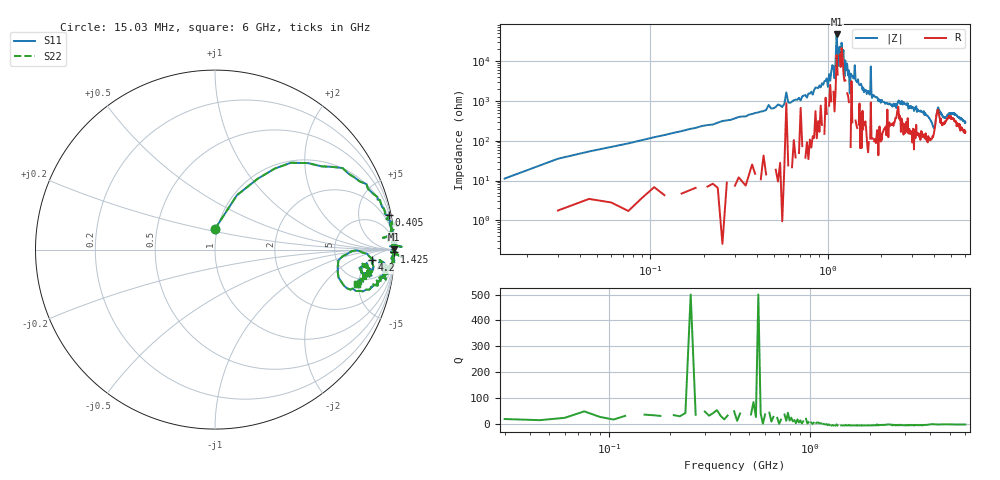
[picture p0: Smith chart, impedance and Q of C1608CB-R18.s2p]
!	Network	Analyzer	HP8753E.07.74:	Oct	30	2002	Serial	No.	JP38451487
!	Hewlett-Packard
!	7	Sep	2009	10:03:13
!	Frequency	S11	S21	S12	S22
#	HZ	S	RI	R	50
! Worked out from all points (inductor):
!   400 points, 15.03 MHz to 6 GHz, reference 50 ohm
!   read as one part in series: L = 184 nH near 45.03 MHz
!   highest |Z| = 45.7 kohm at 1.125 GHz (marker M1)
!   self-resonance near 1.185 GHz
!   S11 on the Smith chart (normalised r, x): 15.03 MHz: 0.97, +0.22; 405 MHz: 1, +10; 1.425 GHz: open; 4.2 GHz: 12, -6; 6 GHz: 4.26, -4.71
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1.502992e7  -0.00146 0.113  1 -0.113  1 -0.113  -0.00146 0.113
9.002955e7  0.518 0.482  0.482 -0.482  0.482 -0.482  0.518 0.482
4.05028e8  0.967 0.191  0.0333 -0.191  0.0333 -0.191  0.967 0.191
1.020025e9  0.996 0.0209  0.00382 -0.0209  0.00382 -0.0209  0.996 0.0209
1.095025e9  0.995 0.0268  0.00473 -0.0268  0.00473 -0.0268  0.995 0.0268
1.125024e9  0.999 0.00208  0.000672 -0.00208  0.000672 -0.00208  0.999 0.00208
1.155024e9  1 0.0134  3.1e-05 -0.0134  3.1e-05 -0.0134  1 0.0134
1.185024e9  0.986 0.000274  0.0139 -0.000274  0.0139 -0.000274  0.986 0.000274
1.200024e9  0.997 -0.00235  0.00262 0.00235  0.00262 0.00235  0.997 -0.00235
1.245024e9  0.98 -0.0148  0.0198 0.0148  0.0198 0.0148  0.98 -0.0148
1.320023e9  0.997 -0.0171  0.00308 0.0171  0.00308 0.0171  0.997 -0.0171
1.335023e9  1.05 -0.0452  -0.0524 0.0452  -0.0524 0.0452  1.05 -0.0452
1.425023e9  1 -0.0129  -0.00097 0.0129  -0.00097 0.0129  1 -0.0129
1.725021e9  0.998 -0.0698  0.00192 0.0698  0.00192 0.0698  0.998 -0.0698
1.755021e9  0.998 -0.0137  0.00192 0.0137  0.00192 0.0137  0.998 -0.0137
1.785021e9  0.985 -0.0832  0.0151 0.0832  0.0151 0.0832  0.985 -0.0832
2.01002e9  0.977 -0.0947  0.0234 0.0947  0.0234 0.0947  0.977 -0.0947
3.015015e9  0.963 -0.134  0.0366 0.134  0.0366 0.134  0.963 -0.134
4.00501e9  0.684 -0.127  0.316 0.127  0.316 0.127  0.684 -0.127
4.200009e9  0.875 -0.0586  0.125 0.0586  0.125 0.0586  0.875 -0.0586
5.010005e9  0.852 -0.0962  0.148 0.0962  0.148 0.0962  0.852 -0.0962
6e9  0.789 -0.189  0.211 0.189  0.211 0.189  0.789 -0.189
